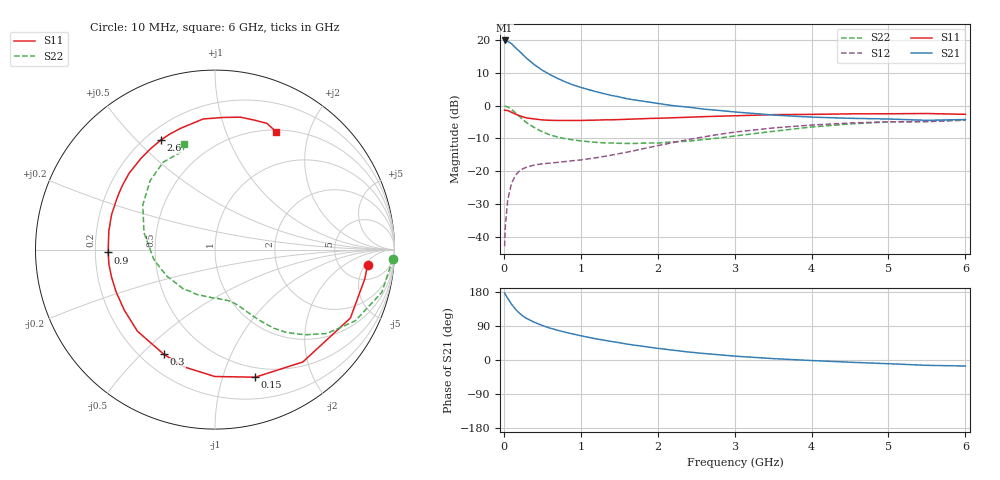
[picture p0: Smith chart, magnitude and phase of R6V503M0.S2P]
! SIEMENS Small Signal Semiconductors
! BFR193
! Si NPN RF Bipolar Junction Transistor in SOT23
! VCE = 0.5 V  IC = 3 mA
! Common Emitter S-Parameters:  May  1996
# GHz  S  MA  R  50
!  f  S11  S21  S12  S22
! GHz  MAG  ANG  MAG  ANG  MAG  ANG  MAG  ANG
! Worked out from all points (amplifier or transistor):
!   36 points, 10 MHz to 6 GHz, reference 50 ohm
!   highest |S21| = 19.9 dB at 10 MHz (marker M1)
!   |S21| within 3 dB of that: start of sweep to 188.6 MHz
!   unconditionally stable (mu >= 1): 983.2 MHz to 2.444 GHz; 5.16 GHz to end of sweep
!   at 250 MHz: K = 0.32, MSG = 17.4 dB, |S12| = -19.2 dB
!   at 1.4 GHz: K = 1.13, MAG = 6.9 dB, |S12| = -15.1 dB
!   at 6 GHz: K = 1.01, MAG = -0.6 dB, |S12| = -4.4 dB
!   S11 on the Smith chart (normalised r, x): 10 MHz: 9, -6; 150 MHz: 0.40, -1.28; 300 MHz: 0.29, -0.59; 900 MHz: 0.25, -0.01; 2.6 GHz: 0.26, +0.59; 6 GHz: 0.52, +1.52
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0.01  0.8545 -5.6  9.902 176.8  0.0072 85.6  0.9917 -3.0
0.02  0.8506 -11.0  9.739 173.0  0.0146 84.3  0.9803 -5.9
0.05  0.8453 -26.8  9.568 162.9  0.0363 75.4  0.9594 -14.4
0.1  0.7947 -52.0  8.858 147.4  0.0656 63.3  0.876 -27.0
0.15  0.7454 -72.5  7.712 134.3  0.0864 53.7  0.7785 -36.9
0.2  0.707 -90.1  6.816 124.1  0.1005 47.0  0.6897 -43.5
0.25  0.6756 -104.9  5.966 115.6  0.1097 41.7  0.6087 -49.3
0.3  0.6493 -116.0  5.242 109.2  0.116 38.4  0.5469 -53.2
0.4  0.6273 -133.5  4.202 99.3  0.1248 34.4  0.4617 -58.1
0.5  0.6077 -146.3  3.481 91.1  0.1299 32.4  0.401 -61.9
0.6  0.5991 -157.2  2.987 84.2  0.1332 32.1  0.359 -65.2
0.7  0.5964 -165.3  2.608 78.4  0.1368 32.6  0.3329 -68.1
0.9  0.5955 -178.5  2.078 68.5  0.1451 34.5  0.3009 -73.4
1.1  0.6 170.3  1.764 59.8  0.1548 38.0  0.2834 -80.5
1.3  0.6084 161.0  1.53 52.3  0.1684 41.4  0.2707 -88.0
1.6  0.621 149.1  1.278 42.0  0.1959 45.4  0.2659 -100.6
2.2  0.6552 128.8  1.002 25.9  0.274 46.7  0.2815 -129.0
2.6  0.6813 116.2  0.887 17.2  0.3348 43.3  0.3047 -150.4
3.5  0.7308 95.2  0.721 3.7  0.4581 29.1  0.4067 166.6
4.5  0.7512 79.1  0.643 -5.9  0.5449 12.4  0.5277 133.2
5.5  0.7603 67.6  0.599 -14.1  0.5703 -2.8  0.5774 107.9
6  0.7393 62.5  0.615 -15.8  0.6009 -7.2  0.6144 106.3
